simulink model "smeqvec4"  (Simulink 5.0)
settings: Solver=ode45  StartTime=0.0  StopTime=60  MaxStep=.05  RelTol=1e-4  AbsTol=1e-4
InitFcn:
  | smvecdef3
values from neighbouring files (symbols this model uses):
  Bm = 0.10    (= 0.1)    [IMabc2.m]    (also in imabcparam.m = 0.01; IMabcrun0.m = 0.01; IMabcrun1.m = 0.001; IMcur0.m = 1e-06)
  H = 0.60    (= 0.6)    [IMabc2.m]    (also in IMcur0.m = 0.3; imdef0vec.m = 0.3; imdef1vec.m = 0.3; imdef2vec.m = 0.3)
  n0 = 0.98    [imdef0vec.m]    (also in imdef1vec.m = 0.978; imdef2vec.m; imdefrotflux.m; imdefSIvec1.m = 0.95)
  Ra = .95    (= 0.95)    [altwdgs.m]    (also in Ccurverun.m = 0.018)
  V = [Vas 0 0].'    [Actac.m]    (also in acttrcalc1.m = str2num(get(h,'string')); im3d.m = eval(get(hVs,'String')); IMabc2.m = [vas vbs vcs 0 0 0]'; IMabcf0.m = [vas vbs vcs 0 0 0]')
  wo = 2*pi*freq0    [calc0.m]    (also in IMabc2.m = 376.991118431; imabcparam.m = 376.991118431; IMabcrun0.m = 376.991118431; IMabcrun1.m = 376.991118431)
undefined symbols (not defined in the file or in its folder): delta0, fa0, fk0, L_1, phif0, Rf, Rkd, Rkq, vf0
libraries: simulink x3

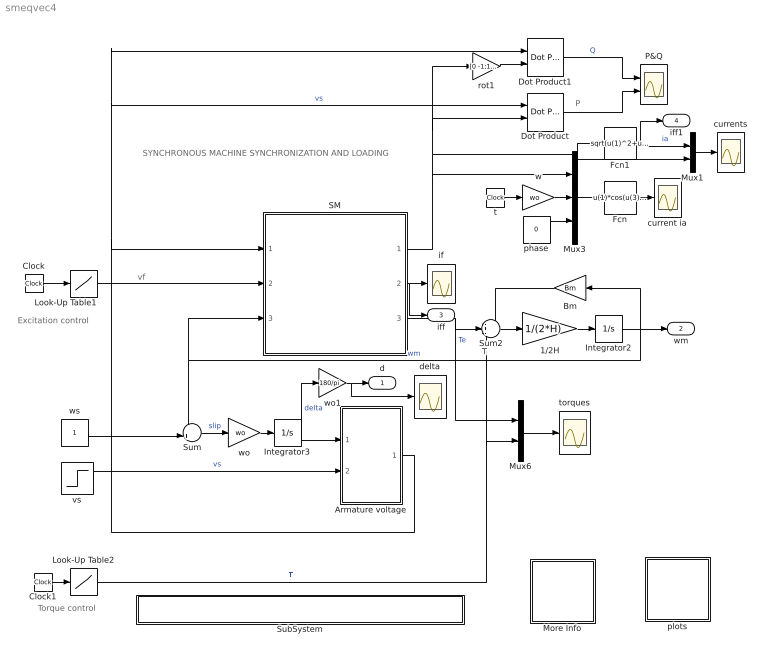
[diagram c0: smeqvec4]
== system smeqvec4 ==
  note: Tl
  note: P
  note: Excitation control
  note: Torque control
  note: SYNCHRONOUS MACHINE SYNCHRONIZATION AND LOADING
  note: vf
  1/2H : Gain  Gain=1/(2*H)
  Armature voltage : Subsystem
  Bm : Gain  Orientation=left  Gain=Bm
  Clock : Clock
  Clock1 : Clock
  Dot Product : simulink/Math Operations/Dot Product
  Dot Product1 : simulink/Math Operations/Dot Product
  Fcn : Fcn  Expr=u(1)*cos(u(3)+u(4))+u(2)*sin(u(3)+u(4))
  Fcn1 : Fcn  Expr=sqrt(u(1)^2+u(2)^2)
  Integrator2 : Integrator  InitialCondition=n0
  Integrator3 : Integrator  InitialCondition=delta0
  Look-Up Table1 : Lookup  InputValues="[0  20  30 50 60]"  OutputValues=[vf0 vf0 .5*vf0 3*vf0 3*vf0]
  Look-Up Table2 : Lookup  InputValues="[0  10  15 100]"  OutputValues=[0 0 -0.82 -.82]
  More Info : Subsystem
  Mux1 : Mux  Inputs=2
  Mux3 : Mux  Inputs=3
  Mux6 : Mux  Inputs=2
  P&Q : Scope  NumInputPorts=2
  SM : Subsystem
  SubSystem : Subsystem
  Sum : Sum  Inputs=-+|
  Sum2 : Sum  Inputs=-+-
  current ia : Scope
  currents : Scope
  delta : Scope
  if : Scope
  phase : Constant  Value=0
  plots : Subsystem
  rot1 : Gain  Gain=[0 -1;1 0]  Multiplication=Matrix(K*u)
  t : Clock
  torques : Scope
  vs : Step  Time=0  After=V  SampleTime=0
  w : Gain  Gain=wo
  wo : Gain  Gain=wo
  wo1 : Gain  Gain=180/pi
  ws : Constant
  d : Outport
  wm : Outport  Port=2
  iff : Outport  Port=3
  iff1 : Outport  Port=4
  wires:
  1/2H/1 -> Integrator2/1
  Sum2/1 -> 1/2H/1
  Bm/1 -> Sum2/1
  SM/3(Te) -> Mux6/1, Sum2/2  "Te"
  Mux6/1 -> torques/1
  SM/1(ia) -> Mux3/1, Dot Product/2, rot1/1, Fcn1/1, Mux1/2
  SM/2(if) -> if/1, iff/1
  Integrator2/1 -> Bm/1, Sum/1, SM/3(wm), wm/1  "wm"
  w/1 -> Mux3/2
  phase/1 -> Mux3/3
  Mux3/1 -> Fcn/1
  t/1 -> w/1
  ws/1 -> Sum/2
  Sum/1 -> wo/1  "slip"
  Armature voltage/1(vs) -> SM/1(vs), Dot Product/1, Dot Product1/1  "vs"
  wo/1 -> Integrator3/1
  vs/1 -> Armature voltage/2(Vt)  "vs"
  Integrator3/1 -> Armature voltage/1(delta), wo1/1  "delta"
  Dot Product/1 -> P&Q/2
  Dot Product1/1 -> P&Q/1  "Q"
  rot1/1 -> Dot Product1/2
  Clock/1 -> Look-Up Table1/1
  Look-Up Table1/1 -> SM/2(vf)
  Clock1/1 -> Look-Up Table2/1
  Fcn1/1 -> iff1/1, Mux1/1  "ia"
  Look-Up Table2/1 -> Mux6/2, Sum2/3  "Tl"
  Fcn/1 -> current ia/1
  Mux1/1 -> currents/1
  wo1/1 -> delta/1, d/1

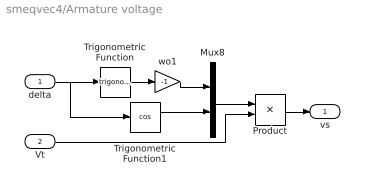
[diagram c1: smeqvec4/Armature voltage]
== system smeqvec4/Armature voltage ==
  delta : Inport
  Vt : Inport  Port=2
  Mux8 : Mux  Inputs=2
  Product : Product
  Trigonometric Function : Trigonometry
  Trigonometric Function1 : Trigonometry  Operator=cos
  wo1 : Gain  Gain=-1
  vs : Outport
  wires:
  delta/1 -> Trigonometric Function/1, Trigonometric Function1/1
  Trigonometric Function/1 -> wo1/1
  Mux8/1 -> Product/1
  wo1/1 -> Mux8/1
  Trigonometric Function1/1 -> Mux8/2
  Product/1 -> vs/1
  Vt/1 -> Product/2

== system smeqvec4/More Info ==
  note: SYNCHRONOUS MACHINE AGAINST AN INFINITE BUS
  note: SYNCHRONIZATION AND LOADING

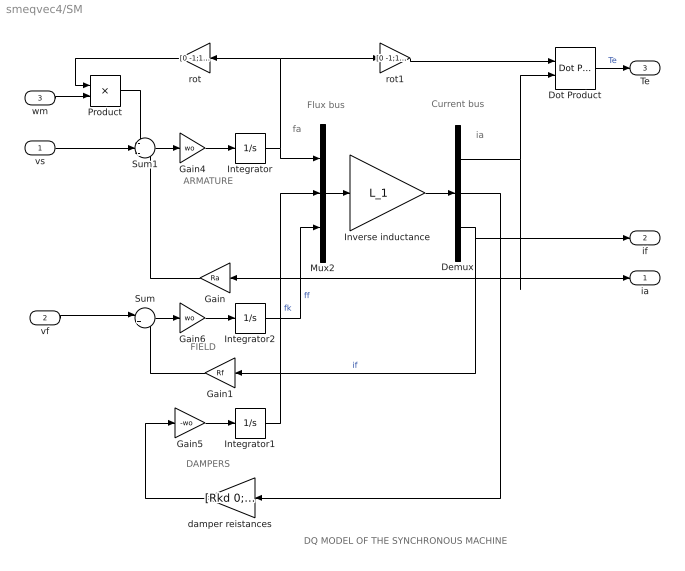
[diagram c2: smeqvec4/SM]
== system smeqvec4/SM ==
  note: DAMPERS
  note: ARMATURE
  note: fa
  note: ia
  note: FIELD
  note: DQ MODEL OF THE SYNCHRONOUS MACHINE
  note: Flux bus
  note: Current bus
  vs : Inport
  vf : Inport  Port=2
  wm : Inport  Port=3
  Demux : Demux  Outputs=3
  Dot Product : simulink/Math Operations/Dot Product
  Gain : Gain  Orientation=left  Gain=Ra
  Gain1 : Gain  Orientation=left  Gain=Rf
  Gain4 : Gain  Gain=wo
  Gain5 : Gain  Gain=-wo
  Gain6 : Gain  Gain=wo
  Integrator : Integrator  InitialCondition=fa0
  Integrator1 : Integrator  InitialCondition=fk0
  Integrator2 : Integrator  InitialCondition=phif0
  Inverse inductance : Gain  Gain=L_1  Multiplication=Matrix(K*u)
  Mux2 : Mux  Inputs=3
  Product : Product
  Sum : Sum  Inputs=|+-
  Sum1 : Sum  Inputs=-+-
  damper reistances : Gain  Orientation=left  Gain=[Rkd 0;0 Rkq]  Multiplication=Matrix(K*u)
  rot : Gain  Orientation=left  Gain=[0 -1;1 0]  Multiplication=Matrix(K*u)
  rot1 : Gain  Gain=[0 -1;1 0]  Multiplication=Matrix(K*u)
  ia : Outport
  if : Outport  Port=2
  Te : Outport  Port=3
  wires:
  Product/1 -> Sum1/1
  rot/1 -> Product/1
  wm/1 -> Product/2
  Gain5/1 -> Integrator1/1
  damper reistances/1 -> Gain5/1
  Integrator/1 -> Mux2/1, rot/1, rot1/1
  Sum1/1 -> Gain4/1
  Gain4/1 -> Integrator/1
  vs/1 -> Sum1/2
  Gain/1 -> Sum1/3
  Gain6/1 -> Integrator2/1
  Sum/1 -> Gain6/1
  vf/1 -> Sum/1
  Gain1/1 -> Sum/2
  rot1/1 -> Dot Product/1
  Demux/1 -> Gain/1, ia/1, Dot Product/2
  Dot Product/1 -> Te/1  "Te"
  Mux2/1 -> Inverse inductance/1
  Inverse inductance/1 -> Demux/1
  Integrator1/1 -> Mux2/2  "fk"
  Integrator2/1 -> Mux2/3  "ff"
  Demux/2 -> damper reistances/1
  Demux/3 -> if/1, Gain1/1  "if"

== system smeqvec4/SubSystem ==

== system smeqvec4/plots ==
